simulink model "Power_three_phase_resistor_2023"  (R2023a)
settings: Solver=VariableStepAuto  StartTime=0.0  StopTime=0.1  MaxStep=1e-5  RelTol=1e-3
libraries: spsACVoltageSourceLib x3, spsSeriesRLCBranchLib x3, spsGroundLib x1, spsPower3phInstantaneousLib x1, spsThreePhaseVIMeasurementLib x1, spspowerguiLib x1

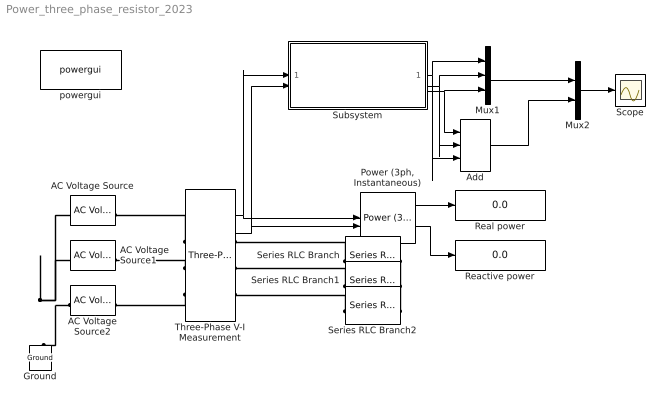
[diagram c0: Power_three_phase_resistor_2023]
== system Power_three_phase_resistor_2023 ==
  AC Voltage Source : spsACVoltageSourceLib/AC Voltage Source  Amplitude=100*sqrt(2)  Phase=0  Frequency=60  SampleTime=0  Measurements=None  BusType=swing  Pref=10e3  Qref=0  Qmin=-inf  Qmax=+inf
  AC Voltage Source1 : spsACVoltageSourceLib/AC Voltage Source  Amplitude=100*sqrt(2)  Phase=-120  Frequency=60  SampleTime=0  Measurements=None  BusType=swing  Pref=10e3  Qref=0  Qmin=-inf  Qmax=+inf
  AC Voltage Source2 : spsACVoltageSourceLib/AC Voltage Source  Amplitude=100*sqrt(2)  Phase=-240  Frequency=60  SampleTime=0  Measurements=None  BusType=swing  Pref=10e3  Qref=0  Qmin=-inf  Qmax=+inf
  Add : Sum  Inputs=+++
  Ground : spsGroundLib/Ground  LConnTagsString=a
  Mux1 : Mux  Inputs=3
  Mux2 : Mux  Inputs=2
  "Power (3ph, Instantaneous)" : spsPower3phInstantaneousLib/Power (3ph, Instantaneous)
  Reactive power : Display
  Real power : Display
  Scope : Scope
  Series RLC Branch : spsSeriesRLCBranchLib/Series RLC Branch  LConnTagsString=__new0  RConnTagsString=__new0  BranchType=R  Resistance=2  Inductance=1e-3  SetiL0=off  InitialCurrent=0  Capacitance=1e-6  Setx0=off  InitialVoltage=0  Measurements=None
  Series RLC Branch1 : spsSeriesRLCBranchLib/Series RLC Branch  LConnTagsString=__new0  RConnTagsString=__new0  BranchType=R  Resistance=2  Inductance=1e-3  SetiL0=off  InitialCurrent=0  Capacitance=1e-6  Setx0=off  InitialVoltage=0  Measurements=None
  Series RLC Branch2 : spsSeriesRLCBranchLib/Series RLC Branch  LConnTagsString=__new0  RConnTagsString=__new0  BranchType=R  Resistance=2  Inductance=1e-3  SetiL0=off  InitialCurrent=0  Capacitance=1e-6  Setx0=off  InitialVoltage=0  Measurements=None
  Subsystem : Subsystem
  Three-Phase V-I Measurement : spsThreePhaseVIMeasurementLib/Three-Phase V-I Measurement  VoltageMeasurement=phase-to-ground  SetLabelV=off  LabelV=Vabc  Vpu=off  VpuLL=off  CurrentMeasurement=yes  SetLabelI=off  LabelI=Iabc  Ipu=off  Pbase=100e6  Vbase=500e3  OutputType=Complex  PhasorSimulation=off  PSBequivalent=0
  powergui : spspowerguiLib/powergui  Priority=1  SimulationMode=Continuous  SampleTime=50e-6  frequency=60  Iterations=50  frequencyindice=60  Pbase=100e6  ErrMax=1e-4  UnitsV=kV  UnitsW=MW  buscounter=0  FunctionMessages=off  echomessages=off  EnableUseOfTLC=off  CurrentSourceSwitches=off  DisableSnubberDevices=off  DisableRonSwitches=off  DisableVfSwitches=off  DisplayEquations=off  AutomaticDiscreteSolvers=off  SolverType=Tustin/Backward Euler (TBE)  Interpol=off  ExternalGateDelay=off  methode=off  Ts=100  x0status=blocks  SPID=on  SwTol=0  HookPort=off  NonlinearTolerance=1e-4  nMaxIteration=100  ContinueOnMaxIteration=off  RestoreLinks=warning  ResistiveCurrentMeasurement=off  Frange=[0:2:500]  Ylog=off  Xlog=on  ShowGrid=off  save=off  variable=ZData  structure=0  ZoomFFT=off  StartTime=0.0  cycles=1  DisplayStyle=1  fundamental=60  FreqAxis=off  MaxFrequency=1000  frequencyindicesteady=1  RmsSteady=1  display=off
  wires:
  Three-Phase V-I Measurement/1 -> Subsystem/1(In1), "Power (3ph, Instantaneous)"/1
  Three-Phase V-I Measurement/2 -> Subsystem/2(In2), "Power (3ph, Instantaneous)"/2
  "Power (3ph, Instantaneous)"/1 -> Real power/1
  "Power (3ph, Instantaneous)"/2 -> Reactive power/1
  Subsystem/1(Pa) -> Add/3, Mux1/1
  Subsystem/2(Pb) -> Add/2, Mux1/2
  Subsystem/3(Pc) -> Add/1, Mux1/3
  Mux1/1 -> Mux2/1
  Add/1 -> Mux2/2
  Mux2/1 -> Scope/1
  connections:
  Three-Phase V-I Measurement/LConn3 -- AC Voltage Source2/RConn1
  Three-Phase V-I Measurement/LConn2 -- AC Voltage Source1/RConn1
  Three-Phase V-I Measurement/LConn1 -- AC Voltage Source/RConn1
  AC Voltage Source2/LConn1 -- AC Voltage Source/LConn1 -- AC Voltage Source1/LConn1 -- Ground/LConn1
  Series RLC Branch/LConn1 -- Three-Phase V-I Measurement/RConn1
  Series RLC Branch1/LConn1 -- Three-Phase V-I Measurement/RConn2
  Series RLC Branch2/LConn1 -- Three-Phase V-I Measurement/RConn3
  Series RLC Branch/RConn1 -- Series RLC Branch1/RConn1 -- Series RLC Branch2/RConn1

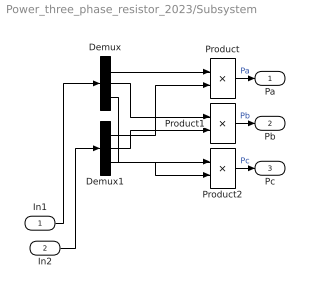
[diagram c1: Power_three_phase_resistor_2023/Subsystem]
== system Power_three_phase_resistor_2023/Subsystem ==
  In1 : Inport
  In2 : Inport  Port=2
  Demux : Demux  Outputs=3
  Demux1 : Demux  Outputs=3
  Product : Product
  Product1 : Product
  Product2 : Product
  Pa : Outport
  Pb : Outport  Port=2
  Pc : Outport  Port=3
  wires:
  In1/1 -> Demux/1
  Demux/1 -> Product/1
  In2/1 -> Demux1/1
  Demux/3 -> Product2/1
  Demux/2 -> Product1/1
  Demux1/3 -> Product2/2
  Demux1/2 -> Product1/2
  Demux1/1 -> Product/2
  Product/1 -> Pa/1  "Pa"
  Product1/1 -> Pb/1  "Pb"
  Product2/1 -> Pc/1  "Pc"
